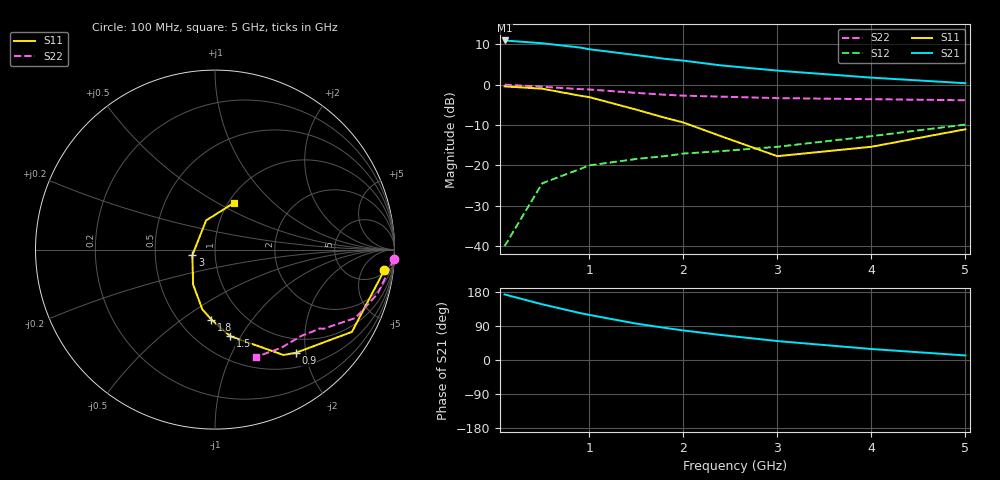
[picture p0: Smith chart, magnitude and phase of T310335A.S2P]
!AT-31033
!S and NOISE PARAMETERS at Vce=5V  Ic=1mA.  LAST UPDATED 06-23-94
# ghz s ma r 50
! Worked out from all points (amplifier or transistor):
!   11 points, 100 MHz to 5 GHz, reference 50 ohm
!   highest |S21| = 10.9 dB at 100 MHz (marker M1)
!   |S21| within 3 dB of that: start of sweep to 1.285 GHz
!   unconditionally stable (mu >= 1): 2.322 GHz to 4.128 GHz
!   at 500 MHz: K = 0.26, MSG = 17.3 dB, |S12| = -24.4 dB
!   at 1.8 GHz: K = 0.86, MSG = 12.1 dB, |S12| = -17.7 dB
!   at 5 GHz: K = 0.90, MSG = 5.1 dB, |S12| = -9.9 dB
!   lowest NFmin = 0.50 dB at 500 MHz
!   S11 on the Smith chart (normalised r, x): 100 MHz: 6, -14; 900 MHz: 0.74, -1.81; 1.5 GHz: 0.71, -0.90; 1.8 GHz: 0.71, -0.65; 3 GHz: 0.77, -0.05; 5 GHz: 1.06, +0.60
0.1  0.95 -7.0  3.52 173.0  0.01 85.0  0.999 -3.0
0.5  0.89 -31.0  3.25 147.0  0.06 70.0  0.94 -15.0
0.9  0.73 -52.0  2.88 124.0  0.09 59.0  0.88 -24.0
1  0.7 -57.0  2.74 119.0  0.1 57.0  0.87 -26.0
1.5  0.49 -80.0  2.32 96.0  0.12 49.0  0.79 -32.0
1.8  0.39 -93.0  2.09 85.0  0.13 47.0  0.75 -36.0
2  0.34 -102.0  1.98 78.0  0.14 46.0  0.73 -37.0
2.4  0.23 -122.0  1.73 66.0  0.15 46.0  0.71 -40.0
3  0.13 -166.0  1.49 50.0  0.17 49.0  0.68 -45.0
4  0.17 107.0  1.22 29.0  0.23 51.0  0.66 -56.0
5  0.28 68.0  1.04 12.0  0.32 48.0  0.64 -69.0
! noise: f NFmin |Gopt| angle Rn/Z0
0.5  0.5  0.9  12  0.7
0.9  0.6  0.82  28  0.6
1.8  1.1  0.57  68  0.38
2.4  1.6  0.41  100  0.22
